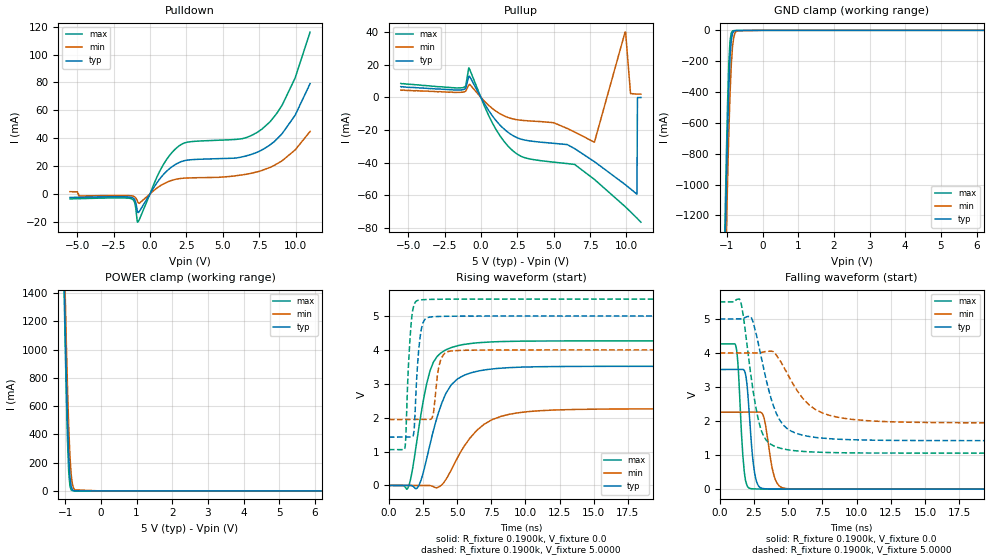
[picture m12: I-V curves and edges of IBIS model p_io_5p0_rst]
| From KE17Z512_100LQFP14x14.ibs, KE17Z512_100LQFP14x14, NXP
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[Model] p_io_5p0_rst
|   Model p_io_5p0_rst
| This model was characterised for following simulation conditions:
| External (pad) voltage:
|   - Typ: 5.0V,   - Min: 4.0V,   - Max: 5.5V
| Library cells for typ/min/max conditions are connected as defined below:
|  pad - External Pad
|  ipp_do_lv - Core Input
|  ipp_obe_lv - Output Buffer Enable
|  abt_close_nor_rst_mv - vdde
|  dvdd - dvdd
|  dvss - dvss
|  esd_boost - vdde
|  ipp_ina_280_mv - NC
|  ipp_ina_40_a_mv - NC
|  ipp_ina_40_b_mv - NC
|  ipp_ina_40_c_mv - NC
|  ipp_ina_40_d_mv - NC
|  ipp_ina_40_e_mv - NC
|  ipp_ina_40_f_mv - NC
|  ipp_ina_40_g_mv - NC
|  ipp_ina_40_h_mv - NC
|  ipp_ind_lv - NC
|  vdde - vdde
|  vsse - vsse
| All other pins connected to ground
Model_type I/O
Polarity   Non-Inverting
Enable   Active-High
Vinl =   1.5000V
Vinh =   3.5000V
Vmeas =  2.5000V
Cref =   50.0000F
C_comp   1.5413pF   1.4782pF   1.6301pF
[Model Spec]
| variable   typ   min   max
Vinh   3.5000V   2.8000V   3.8500V
Vinl   1.5000V   1.2000V   1.6500V
S_overshoot_high   5.3000V   4.3000V   5.8000V
S_overshoot_low   -0.3000V   -0.3000V   -0.3000V
Vmeas   2.5000V   2.0000V   2.7500V
[Temperature Range]   25.0000   0.1250k   -40.0000
[Voltage Range]   5.0000V   4.0000V   5.5000V
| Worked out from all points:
|   slope of the pulldown table from 0 to 0.75 V, typ, clamps not added: 63.6 ohm
|   slope of the pullup table from 0 to 0.75 V, typ, clamps not added: 69.2 ohm
|   GND clamp passes 1 mA (typ) near -0.73 V on its own axis
|   POWER clamp passes 1 mA (typ) near -0.73 V on its own axis
|   rising waveform, R_fixture 0.1900k, V_fixture 0.0: 20-80 % time 1.61ns typ, 2.43ns min, 1.16ns max; typ from 0 V to 3.52 V
|   rising waveform, R_fixture 0.1900k, V_fixture 5.0000: 20-80 % time 342ps typ, 386ps min, 315ps max; typ from 1.43 V to 5 V
|   falling waveform, R_fixture 0.1900k, V_fixture 0.0: 20-80 % time 421ps typ, 552ps min, 342ps max; typ from 3.52 V to 0 V
|   falling waveform, R_fixture 0.1900k, V_fixture 5.0000: 20-80 % time 1.42ns typ, 2.25ns min, 998ps max; typ from 5 V to 1.43 V
[Pulldown]
|Voltage   I(typ)   I(min)   I(max)
-5.5V     -2.57mA    1.56mA     -3.61mA
-4.888V   -2.45mA    -1.53mA    -3.44mA
-1.318V   -2.427mA   -1.367mA   -3.377mA
-1.046V   -4.365mA   -2.203mA   -6.507mA
-842mV    -13.24mA   -5.799mA   -20.33mA
790mV     12.31mA    6.353mA    18.69mA
1.946V    22.23mA    10.81mA    34.02mA
6.332V    26.55mA    13.6mA     39.6mA
8.236V    35.1mA     18.9mA     51.6mA
9.086V    43.3mA     23.8mA     63.8mA
9.97V     56.4mA     31.5mA     83.1mA
11V       79.1mA     44.8mA     116.1mA
[Pullup]
|Voltage   I(typ)   I(min)   I(max)
-5.5V     6.5mA      4.4mA      8.5mA
-1.24V    4.62mA     3.14mA     5.89mA
-832mV    12.93mA    7.462mA    18.04mA
800mV     -11.48mA   -6.914mA   -15.85mA
2.16V     -23.18mA   -13.13mA   -32.42mA
5.934V    -28.91mA   -19.06mA   -40.55mA
7.804V    -39.38mA   -27.47mA   -50.26mA
9.912V    -53.35mA   39.94mA    -66.86mA
10.29V    -56.05mA   2.32mA     -70.07mA
10.73V    -59.34mA   1.94mA     -73.97mA
10.76V    -130uA     1.94mA     -74.28mA
11V       -120uA     1.95mA     -76.44mA
[GND_clamp]
|Voltage   I(typ)   I(min)   I(max)
-5.5V     -66.62A    -66.5A     -66.75A
-1.08V    -1.774A    -2.076A    -1.597A
-1.046V   -1.369A    -1.681A    -1.183A
-1.012V   -991.6mA   -1.308A    -798.4mA
-978mV    -653.5mA   -965.4mA   -463.8mA
-944mV    -373.9mA   -662.6mA   -209.8mA
-910mV    -174.9mA   -412.7mA   -66.67mA
-876mV    -64.97mA   -227.3mA   -16.28mA
-842mV    -20.54mA   -109.6mA   -4.484mA
-774mV    -2.326mA   -19.13mA   -1.536mA
-706mV    -738.8uA   -3.096mA   -1.054mA
11V       0A         0A         0A
[POWER_clamp]
|Voltage   I(typ)   I(min)   I(max)
-5.5V     71.4A      71.12A     71.63A
-1.036V   1.612A     1.825A     1.497A
-1.002V   1.196A     1.424A     1.067A
-968mV    816.8mA    1.053A     676.5mA
-934mV    491.1mA    724.1mA    351.9mA
-900mV    244.3mA    450.6mA    132.5mA
-866mV    95.52mA    246.8mA    34.14mA
-832mV    30.34mA    117.7mA    7.242mA
-798mV    8.748mA    49.97mA    1.686mA
-730mV    848uA      7.656mA    382.7uA
0V        97.87pA    1.039nA    90.77pA
11V       0A         0A         0A
[Ramp]
| variable   typ   min   max
dV/dt_r  2.1095/1.6066n   1.3562/2.4278n   2.5595/1.1620n
dV/dt_f  2.1448/1.4164n   1.2321/2.2534n   2.6655/0.9977n
R_load = 0.1900k
[Rising Waveform]
R_fixture= 0.1900k
V_fixture= 0.0
V_fixture_min= 0.0
V_fixture_max= 0.0
|time   V(typ)   V(min)   V(max)
0s        1.085nV    12.28nV    7.674nV
1.399ns   -46.44uV   -1.667uV   -70.99mV
2.134ns   -46.04mV   -8.209uV   1.537V
2.757ns   766.3mV    160.2uV    2.979V
3.253ns   1.605V     -34.27mV   3.632V
4.175ns   2.714V     172.4mV    4.001V
4.945ns   3.111V     755.5mV    4.115V
6.981ns   3.406V     1.806V     4.223V
10.13ns   3.496V     2.175V     4.259V
40ns      3.516V     2.26V      4.266V
[Rising Waveform]
R_fixture= 0.1900k
V_fixture= 5.0000
V_fixture_min= 4.0000
V_fixture_max= 5.5000
|time   V(typ)   V(min)   V(max)
0s        1.425V     1.946V     1.058V
1.184ns   1.425V     1.946V     1.12V
1.638ns   1.426V     1.946V     4.812V
1.861ns   1.697V     1.946V     5.348V
2.141ns   3.776V     1.946V     5.464V
2.587ns   4.87V      1.947V     5.483V
3.176ns   4.977V     2.003V     5.492V
3.706ns   4.987V     3.573V     5.495V
4.482ns   4.994V     3.964V     5.497V
40ns      5V         4V         5.5V
[Falling Waveform]
R_fixture= 0.1900k
V_fixture= 0.0
V_fixture_min= 0.0
V_fixture_max= 0.0
|time   V(typ)   V(min)   V(max)
0s        3.516V     2.26V      4.266V
1.196ns   3.515V     2.26V      4.18V
1.75ns    3.508V     2.26V      687.1mV
1.98ns    3.12V      2.26V      120.7mV
2.188ns   2.038V     2.26V      23.73mV
2.725ns   178.1mV    2.262V     5.004mV
3.227ns   14.75mV    2.106V     2.845mV
4.031ns   3.752mV    311.1mV    1.485mV
4.732ns   2.122mV    24.89mV    936.6uV
40ns      144.1nV    373.7nV    76.38nV
[Falling Waveform]
R_fixture= 0.1900k
V_fixture= 5.0000
V_fixture_min= 4.0000
V_fixture_max= 5.5000
|time   V(typ)   V(min)   V(max)
0s        5V         4V         5.5V
1.48ns    5V         4V         5.561V
2.308ns   5.042V     4V         3.255V
2.749ns   4.413V     3.999V     2.176V
3.197ns   3.566V     4.031V     1.566V
3.884ns   2.491V     4.043V     1.284V
4.504ns   1.956V     3.713V     1.194V
6.534ns   1.547V     2.472V     1.097V
9.637ns   1.452V     2.051V     1.066V
40ns      1.425V     1.946V     1.058V
